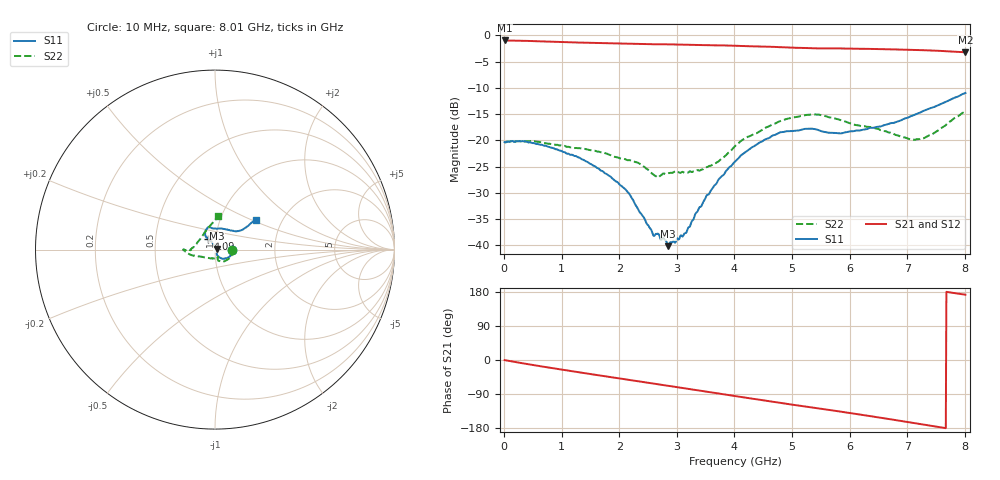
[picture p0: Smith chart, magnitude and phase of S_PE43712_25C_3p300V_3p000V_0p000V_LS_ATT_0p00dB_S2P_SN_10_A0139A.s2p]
! DEVICE ID: PE43712
! File Path: z:\PE43713\PE43713_CHAR_NOM_04292014\AMB\3p300\LS_ATT_0p00dB\PE43713_AMB_3p300V_3p000V_0p000V_LS_ATT_0p00dB_S2P_SN_10_A0139A.s2p
! Serial: 10
! Lot: A0139A
! Temp: 25C
! VDD: 3.300
! VSS: 0.000
! Control_Hi: 3.000
! Control_Lo: 0.000
! Attenuation Step: 0.00dB
! Port 1: RF1
! Port 2: RF2
! ThroughPath:1-2
! IDD: 0.0001467396
! ISS: -1.42e-007
#  Hz  S  RI  R  50
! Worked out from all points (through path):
!   801 points, 10 MHz to 8.01 GHz, reference 50 ohm
!   highest |S21| = -0.95 dB at 10 MHz (marker M1); lowest = -3.2 dB at 8.01 GHz (marker M2)
!   group delay of S21, straight-line fit = 64.2 ps
!   lowest |S11| = -40.2 dB at 2.85 GHz (marker M3), VSWR 1.02, Z = 50.9 + j0.464 ohm
!   |S11| at or under -10 dB: start of sweep to end of sweep
!   |S22| runs from -27.1 to -14.5 dB; largest |S21 - S12| = 0.003
!   S11 on the Smith chart (normalised r, x): 10 MHz: 1.21, -0.00; 4.09 GHz: 0.92, +0.11; 8.01 GHz: 1.47, +0.54
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1e7  0.0962 -0.000619  0.8963 -0.00472  0.896 -0.00437  0.0961 -0.000995
3.6e8  0.0944 -0.0245  0.8749 -0.1467  0.8773 -0.1461  0.0936 -0.0257
6.9e8  0.0801 -0.0392  0.8347 -0.2693  0.8342 -0.2692  0.084 -0.0429
1.35e9  0.0424 -0.0506  0.7119 -0.4729  0.7114 -0.4726  0.0524 -0.0649
1.82e9  0.0219 -0.0406  0.6018 -0.5896  0.6014 -0.5893  0.0326 -0.0655
2.09e9  0.0122 -0.0326  0.5307 -0.6473  0.5304 -0.6468  0.0201 -0.0633
2.34e9  0.00924 -0.0192  0.46 -0.693  0.4599 -0.6927  0.0164 -0.0582
2.58e9  0.0115 -0.00587  0.3883 -0.7275  0.3886 -0.7276  0.0132 -0.0459
2.68e9  0.0128 -0.000153  0.36 -0.7408  0.3602 -0.7404  0.0166 -0.0412
2.85e9  0.00867 0.00456  0.3073 -0.7626  0.3074 -0.7627  0.00932 -0.0478
3.14e9  0.000641 0.013  0.2137 -0.7891  0.2139 -0.7887  -0.0059 -0.0486
3.36e9  -0.00441 0.0206  0.1413 -0.7991  0.1416 -0.7994  -0.0164 -0.0494
3.69e9  -0.013 0.0366  0.0337 -0.8046  0.0344 -0.805  -0.0405 -0.0461
4.01e9  -0.0316 0.054  -0.0712 -0.7952  -0.0705 -0.7948  -0.0787 -0.0396
4.09e9  -0.0371 0.0587  -0.0976 -0.7892  -0.0967 -0.7894  -0.0884 -0.0382
4.78e9  -0.0536 0.1057  -0.3004 -0.7127  -0.2998 -0.713  -0.15 -0.022
5.35e9  -0.0343 0.1246  -0.4377 -0.6169  -0.4375 -0.616  -0.1775 -0.00139
5.85e9  0.00963 0.1162  -0.5453 -0.5184  -0.5439 -0.5186  -0.1553 -0.00148
6.68e9  0.0981 0.1048  -0.6726 -0.3029  -0.6725 -0.3023  -0.1178 0.0154
7.06e9  0.1338 0.1043  -0.7062 -0.1897  -0.7055 -0.1897  -0.0888 0.0501
7.26e9  0.1532 0.11  -0.7135 -0.1277  -0.7126 -0.1274  -0.0696 0.0771
8.01e9  0.2279 0.1673  -0.685 0.0925  -0.6826 0.0912  0.0181 0.1883
